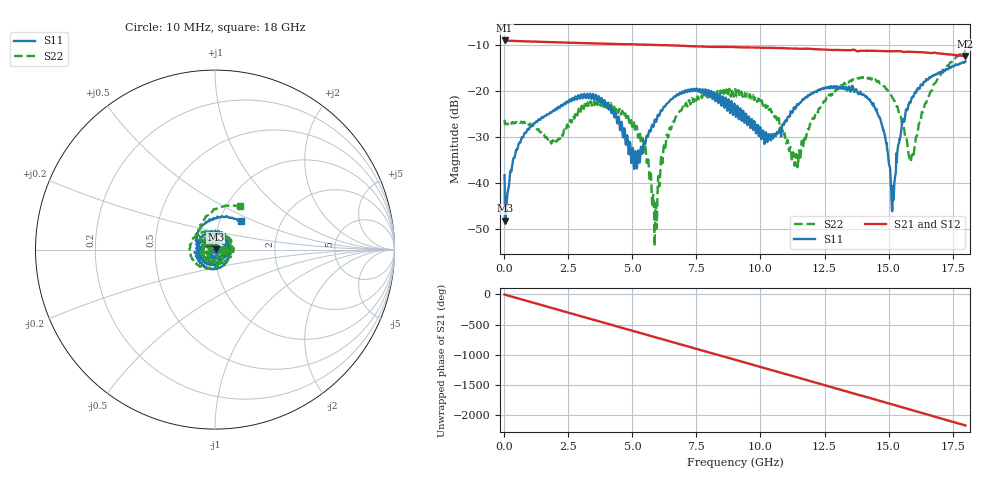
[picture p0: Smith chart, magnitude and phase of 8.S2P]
!Agilent Technologies,E5071C,MY46316741,A.11.02
!Date: Tue Sep 22 10:34:36 2020
!Data & Calibration Information:
!Freq	S11:SOLT4(ON)	S21:SOLT4(ON)	S12:SOLT4(ON)	S22:SOLT4(ON)
!PortZ  Port1:50+j0  Port2:50+j0
!Above PortZ is port z conversion or system Z0 setting when saving the data.
!When reading, reference impedance value at option line is always used.
# Hz S dB R 50
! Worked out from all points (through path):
!   1561 points, 10 MHz to 18 GHz, reference 50 ohm
!   highest |S21| = -8.91 dB at 10 MHz (marker M1); lowest = -12.3 dB at 18 GHz (marker M2)
!   group delay of S21, straight-line fit = 334 ps
!   lowest |S11| = -48.1 dB at 33.06 MHz (marker M3), VSWR 1.01, Z = 50.4 + j0.165 ohm
!   |S11| at or under -10 dB: start of sweep to end of sweep
!   |S22| runs from -53.6 to -11.0 dB; largest |S21 - S12| = 0.0094
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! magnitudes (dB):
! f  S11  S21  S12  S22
! 10 MHz  -38.2  -8.9  -8.9  -26.1
! 33.06 MHz  -48.1  -8.9  -8.9  -27.1
! 851.8 MHz  -29.0  -9.1  -9.1  -26.9
! 1.994 GHz  -23.8  -9.3  -9.3  -31.0
! 3.02 GHz  -20.8  -9.5  -9.5  -23.1
! 4.069 GHz  -23.9  -9.6  -9.7  -22.8
! 5.119 GHz  -33.0  -9.8  -9.8  -28.7
! 5.557 GHz  -29.6  -9.8  -9.8  -35.5
! 5.88 GHz  -26.1  -9.9  -9.9  -48.9
! 6.007 GHz  -25.1  -9.9  -9.9  -38.6
! 6.283 GHz  -23.2  -9.9  -10.0  -32.3
! 6.906 GHz  -20.5  -10.1  -10.1  -24.2
! 9.005 GHz  -23.3  -10.4  -10.4  -19.7
! 10.33 GHz  -29.3  -10.5  -10.5  -23.9
! 11.39 GHz  -23.4  -10.7  -10.7  -33.6
! 12.01 GHz  -20.4  -10.8  -10.8  -26.2
! 14.19 GHz  -21.5  -11.1  -11.2  -17.2
! 15 GHz  -35.0  -11.3  -11.3  -20.2
! 15.19 GHz  -43.6  -11.3  -11.3  -21.7
! 15.87 GHz  -22.2  -11.4  -11.4  -35.3
! 16.8 GHz  -16.4  -11.6  -11.7  -18.2
! 18 GHz  -13.5  -12.3  -12.4  -11.0
